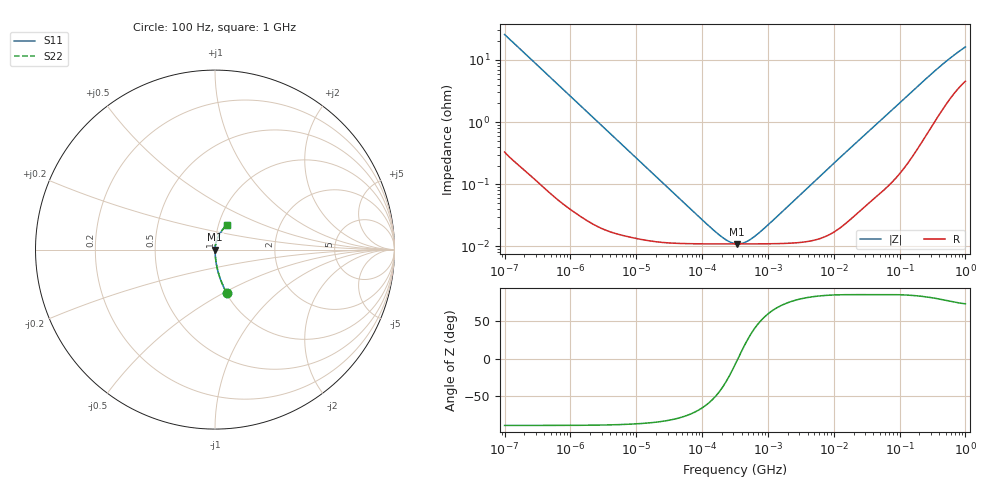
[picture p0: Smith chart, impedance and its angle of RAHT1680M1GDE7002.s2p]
! RAHT1680M1GDE7002  S-PARAMETER MODEL  (AEC-Q200 qualified)
! Model Generated by ELNA Corporation (http://www.ty-top.com)
! Version 1.0
! ELNA Control No. 240229
! Copyright (c) 2024 ELNA CO.,LTD. All Rights Reserved.
! Products Name : CONDUCTIVE POLYMER HYBRID ALUMINUM ELECTROLYTIC CAPACITORS
! Characteristics :
!  Capacitance  :  68uF  ,  Rated voltage  :  35V
!  Operating Temp. Range  :  -55 to +105 degC  ,  Endurance  :  5000hr at 105 degC
!  Dimension D  :  6.3mm  ,  Dimension L  :  7.7mm
! Frequency Range : 100Hz - 1GHz
! External Node Assignments :
!  1  o---| |---o  2
# MHz S RI R 50
!Freq[MHz].  S11 Real  S11 Imag  S21 Real  S21 Imag  S12 Real  S12 Imag  S22 Real  S22 Imag
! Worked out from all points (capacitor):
!   401 points, 100 Hz to 1 GHz, reference 50 ohm
!   read as one part in series: C = 61.9 uF near 108 Hz
!   lowest |Z| = 11 mohm at 342.8 kHz (marker M1)
!   series resonance near 349.8 kHz, so ESL is about 3.3 nH
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0.0001  0.0646 -0.2395  0.9354 0.2395  0.9354 0.2395  0.0646 -0.2395
0.000113  0.0518 -0.2154  0.9482 0.2154  0.9482 0.2154  0.0518 -0.2154
0.000183  0.0212 -0.1376  0.9788 0.1376  0.9788 0.1376  0.0212 -0.1376
0.000309  0.00805 -0.083  0.9919 0.083  0.9919 0.083  0.00805 -0.083
0.000613  0.00238 -0.0423  0.9976 0.0423  0.9976 0.0423  0.00238 -0.0423
0.001488  0.000603 -0.0176  0.9994 0.0176  0.9994 0.0176  0.000603 -0.0176
0.022131  0.000119 -0.0012  0.9999 0.0012  0.9999 0.0012  0.000119 -0.0012
0.098288  0.00011 -0.00025  0.9999 0.00025  0.9999 0.00025  0.00011 -0.00025
0.165959  0.00011 -0.000125  0.9999 0.000125  0.9999 0.000125  0.00011 -0.000125
0.238506  0.00011 -5.99e-05  0.9999 5.99e-05  0.9999 5.99e-05  0.00011 -5.99e-05
0.316228  0.00011 -1.54e-05  0.9999 1.54e-05  0.9999 1.54e-05  0.00011 -1.54e-05
0.342768  0.00011 -3.08e-06  0.9999 3.08e-06  0.9999 3.08e-06  0.00011 -3.08e-06
0.402717  0.00011 2.16e-05  0.9999 -2.16e-05  0.9999 -2.16e-05  0.00011 2.16e-05
0.473151  0.00011 4.68e-05  0.9999 -4.68e-05  0.9999 -4.68e-05  0.00011 4.68e-05
0.679986  0.00011 0.000109  0.9999 -0.000109  0.9999 -0.000109  0.00011 0.000109
1.148154  0.00011 0.000227  0.9999 -0.000227  0.9999 -0.000227  0.00011 0.000227
4.704354  0.000125 0.00102  0.9999 -0.00102  0.9999 -0.00102  0.000125 0.00102
69.9842  0.00118 0.0142  0.9988 -0.0142  0.9988 -0.0142  0.00118 0.0142
176.8072  0.00459 0.0349  0.9954 -0.0349  0.9954 -0.0349  0.00459 0.0349
380.1894  0.017 0.0701  0.983 -0.0701  0.983 -0.0701  0.017 0.0701
668.3439  0.0399 0.1079  0.9601 -0.1079  0.9601 -0.1079  0.0399 0.1079
1000  0.0642 0.1393  0.9358 -0.1393  0.9358 -0.1393  0.0642 0.1393
